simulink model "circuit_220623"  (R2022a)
settings: Solver=VariableStepAuto  StartTime=-D+0.1e-6  StopTime=34e-6  FixedStep=1e-3  MaxStep=0.1e-6  RelTol=1e-3
model workspace (MATLAB code in the model file):
  sGeo = CreateGeometry()
  sConst = CreateConstants()
libraries: fl_lib x9, nesl_utility x3, ee_lib x1

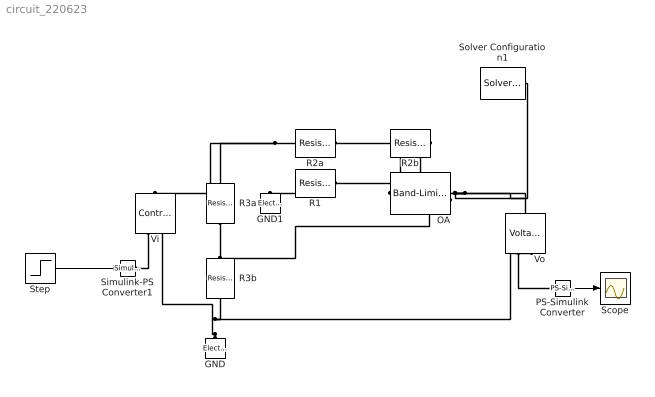
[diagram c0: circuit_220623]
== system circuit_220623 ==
  GND : fl_lib/Electrical/Electrical Elements/Electrical Reference
  GND1 : fl_lib/Electrical/Electrical Elements/Electrical Reference
  OA : ee_lib/Integrated Circuits/Band-Limited Op-Amp  A=100000  Rin=1e8 Ohm  Rout=0 Ohm  Vmin=-15 V  Vmax=15 V  Vdotmax=1000000 V/s  f=10 Hz  V0=0 V
  PS-Simulink Converter : nesl_utility/PS-Simulink Converter  PhysicalDomain=network_engine_domain  SubClassName=ps_output  LeftPortType=input  RightPortType=output  PseudoPeriodic=off  Frequencies=[]  VectorFormat=1-D array  Unit=inherit  AffineConversion=off
  R1 : fl_lib/Electrical/Electrical Elements/Resistor  R=100 kOhm  i_specify=off  i_priority=None  i=0 A  i_nominal_specify=off  i_nominal_unit=A  i_nominal_value=1  v_specify=off  v_priority=None  v=0 V  v_nominal_specify=off  v_nominal_unit=V  v_nominal_value=1
  R2a : fl_lib/Electrical/Electrical Elements/Resistor  R=200 kOhm  i_specify=off  i_priority=None  i=0 A  i_nominal_specify=off  i_nominal_unit=A  i_nominal_value=1  v_specify=off  v_priority=None  v=0 V  v_nominal_specify=off  v_nominal_unit=V  v_nominal_value=1
  R2b : fl_lib/Electrical/Electrical Elements/Resistor  R=200 kOhm  i_specify=off  i_priority=None  i=0 A  i_nominal_specify=off  i_nominal_unit=A  i_nominal_value=1  v_specify=off  v_priority=None  v=0 V  v_nominal_specify=off  v_nominal_unit=V  v_nominal_value=1
  R3a : fl_lib/Electrical/Electrical Elements/Resistor  R=2 kOhm  i_specify=off  i_priority=None  i=0 A  i_nominal_specify=off  i_nominal_unit=A  i_nominal_value=1  v_specify=off  v_priority=None  v=0 V  v_nominal_specify=off  v_nominal_unit=V  v_nominal_value=1
  R3b : fl_lib/Electrical/Electrical Elements/Resistor  R=2 kOhm  i_specify=off  i_priority=None  i=0 A  i_nominal_specify=off  i_nominal_unit=A  i_nominal_value=1  v_specify=off  v_priority=None  v=0 V  v_nominal_specify=off  v_nominal_unit=V  v_nominal_value=1
  Scope : Scope
  Simulink-PS Converter1 : nesl_utility/Simulink-PS Converter  PhysicalDomain=network_engine_domain  SubClassName=ps_input  LeftPortType=input  RightPortType=output  PseudoPeriodic=off  Frequencies=[]  NoiseDistribution=none  NoiseParameters=[]  Unit=1  AffineConversion=off  FilteringAndDerivatives=provide  SimscapeFilterOrder=1  InputFilterTimeConstant=0.001  UdotUserProvided=0
  Solver Configuration1 : nesl_utility/Solver Configuration  PhysicalDomain=network_engine_domain  SubClassName=solver  LeftPortType=input  RightPortType=generic  Tones=[]  Harmonics=[]  SimulateNoise=off  Profile=off  UseLocalSampling=off  EnableSwitchedLinearOptims=on  FrequencyDomain=off  UseCCode=off  RelTol=0.001  AbsTol=1e-06  MinStep=1e-09  ToWorkspace=off  RevertToSquareIcSolve=off  NumHomotopyIterations=100  PhasorMode=off  PhasorModeNumHarmonics=1  IndexReductionMethod=DerivativeReplacement  DoDC=off  ResidualTolerance=1e-09  UseLocalSolver=off  LocalSolverChoice=NE_BACKWARD_EULER_ADVANCER  LocalSolverSampleTime=0.001  DoFixedCost=off  MaxNonlinIter=3  MaxModeIter=2  ComputeImpulses=off  ImpulseIterations=2  LinearAlgebra=Sparse  LinearAlgebraNumThread=0  EquationFormulation=NE_TIME_EF  DelaysMemoryBudget=1024  AutomaticFiltering=on  FilteringTimeConstant=0.001  PartitionStorageMethod=AS_NEEDED  PartitionMemoryBudget=1024  PartitionMethod=FAST
  Step : Step  SampleTime=0
  Vi : fl_lib/Electrical/Electrical Sources/Controlled Voltage Source
  Vo : fl_lib/Electrical/Electrical Sensors/Voltage Sensor
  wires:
  Step/1 -> Simulink-PS Converter1/1
  PS-Simulink Converter/1 -> Scope/1
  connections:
  Vo/RConn1 -- PS-Simulink Converter/LConn1
  OA/RConn1 -- R2b/LConn1 -- Solver Configuration1/RConn1 -- Vo/LConn1
  GND/LConn1 -- R3b/LConn1 -- Vo/RConn2 -- Vi/RConn2
  R2b/RConn1 -- OA/LConn2 -- R1/LConn1 -- R2a/LConn1
  Vi/RConn1 -- Simulink-PS Converter1/RConn1
  R2a/RConn1 -- R3a/RConn1 -- Vi/LConn1
  R1/RConn1 -- GND1/LConn1
  R3b/RConn1 -- OA/LConn1 -- R3a/LConn1
